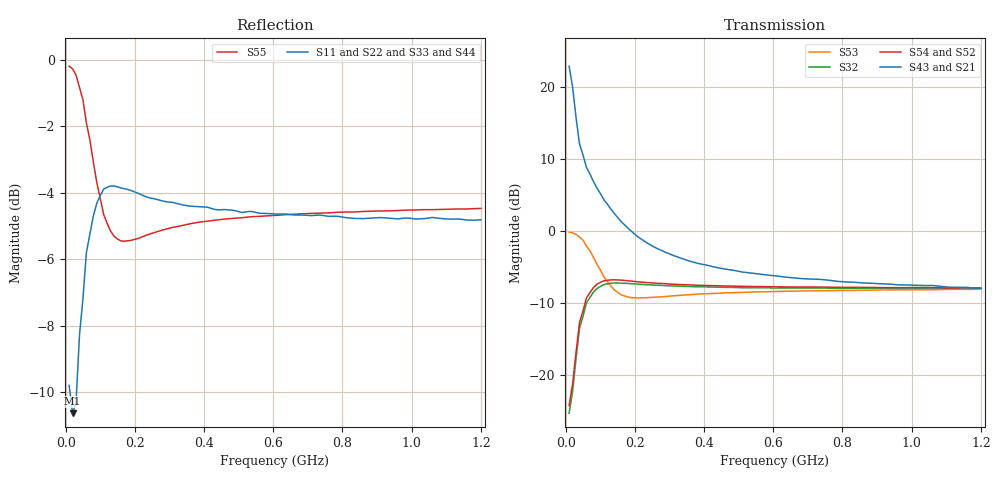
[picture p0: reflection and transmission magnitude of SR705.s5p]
!  POLYFET RF DEVICES
!  S PARAMETERS FOR
!  SR705 (EACH SIDE)
!  VDS=28, IDQ=600MA
! Date: Tue May 11 11:32:10 1999
!AWR Design Environment (2053) Wed Feb 04 15:42:33 2004
!freq-unit  param-type  data-format  keyword  impedance-ohms
# MHz  S  MA  R  50
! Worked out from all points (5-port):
!   120 points, 10 MHz to 1.2 GHz, reference 50 ohm
!   strongest paths, dB at 10 MHz, 310 MHz, 610 MHz, 910 MHz, 1.2 GHz:
!     S43: 22.8, -3.4, -6.2, -7.3, -8.0
!     S21: 22.8, -3.4, -6.2, -7.3, -8.0
!     S54: -24.2, -7.4, -7.7, -7.8, -7.9
!     S52: -24.2, -7.4, -7.7, -7.8, -7.9
!     S32: -25.3, -7.6, -7.9, -7.9, -7.9
!     S53: -0.2, -9.0, -8.4, -8.2, -8.1
!   lowest |S11| = -10.6 dB at 20 MHz (marker M1), VSWR 1.83, Z = 50.5 - j30.9 ohm
!   |S11| at or under -10 dB: 12.36 MHz to 31.58 MHz (19.22 MHz wide, 87.5 % of centre)
